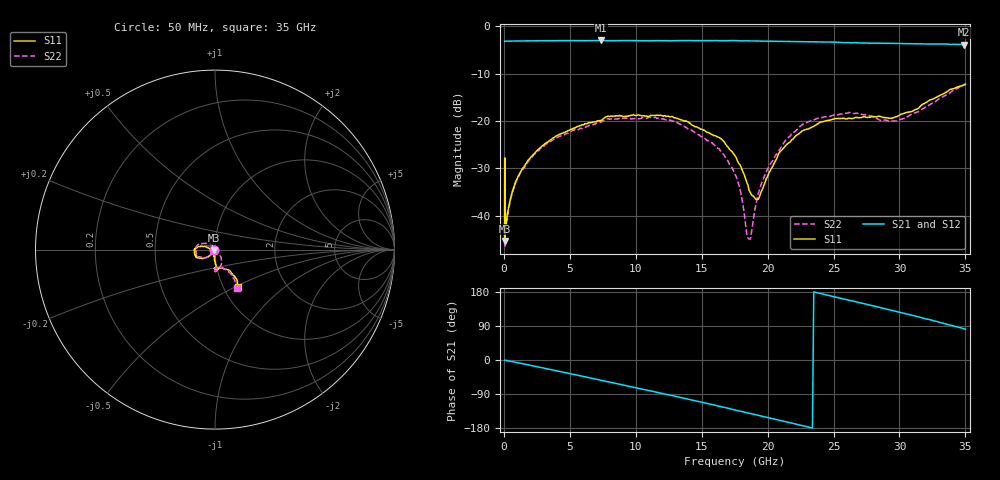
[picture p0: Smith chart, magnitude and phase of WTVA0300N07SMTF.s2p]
! 50 ohm 2-Port S-parameters measured by Modelithics Inc support@modelithics.com  Tampa, FL USA 813-866-6335 (February 2024)
! Smiths Interconnect,  3dB P/N: WTVA0300N07SMTF, Temperature: 25C
! Board: 10 mil Rogers 4350B, Mounting Pad Dimensions: Length: 15 mils, Width: 25 mils, Gap: 40 mils.
# Hz S MA R 50
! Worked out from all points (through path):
!   486 points, 50 MHz to 35 GHz, reference 50 ohm
!   highest |S21| = -2.97 dB at 7.35 GHz (marker M1); lowest = -3.8 dB at 34.9 GHz (marker M2)
!   group delay of S21, straight-line fit = 21.9 ps
!   lowest |S11| = -45.4 dB at 50 MHz (marker M3), VSWR 1.01, Z = 49.5 - j0.282 ohm
!   |S11| at or under -10 dB: start of sweep to end of sweep
!   |S22| runs from -46.5 to -12.2 dB; largest |S21 - S12| = 0.016
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5e7  0.005376 -148.1  0.6975 -0.4  0.6974 -0.4  0.004999 -168.1
8e7  0.006827 -143.7  0.6983 -0.5  0.6975 -0.5  0.004748 -157.2
9e7  0.008086 -161.6  0.6982 -0.6  0.6979 -0.6  0.006899 -158.3
5e8  0.01522 -130.1  0.6993 -3.3  0.699 -3.3  0.01473 -127.3
9e8  0.02285 -127.3  0.7018 -6.1  0.7019 -6.0  0.02237 -125.0
1.95e9  0.04015 -129.9  0.7035 -13.6  0.7034 -13.6  0.03912 -126.7
3.7e9  0.0658 -137.4  0.7066 -26.4  0.7063 -26.4  0.06275 -136.7
5.9e9  0.09124 -148.0  0.7064 -42.5  0.7063 -42.5  0.08326 -148.1
7.35e9  0.1013 -154.4  0.7106 -53.3  0.7105 -53.2  0.09724 -155.5
1.17e10  0.1149 -178.4  0.7067 -86.0  0.7064 -85.8  0.1074 174.1
1.58e10  0.07184 165.2  0.7072 -117.7  0.7075 -117.7  0.05848 142.6
1.76e10  0.04137 165.4  0.7085 -132.6  0.7084 -132.4  0.02614 119.4
1.86e10  0.01841 -176.9  0.7028 -140.5  0.702 -140.4  0.005632 34.1
1.92e10  0.01474 -135.7  0.7008 -145.4  0.7008 -145.3  0.01523 -29.8
2.01e10  0.02829 -97.7  0.6977 -152.6  0.6974 -152.3  0.03356 -47.4
2.12e10  0.05153 -92.9  0.6958 -161.5  0.6955 -161.3  0.05787 -53.0
2.34e10  0.08663 -86.4  0.6887 -179.5  0.689 -179.2  0.1012 -74.9
2.62e10  0.107 -91.9  0.6721 157.6  0.6719 157.7  0.1233 -88.5
2.92e10  0.1068 -75.5  0.663 132.9  0.6631 133.4  0.09943 -84.4
3.19e10  0.1534 -54.7  0.6515 109.3  0.6513 110.5  0.1377 -58.7
3.49e10  0.2406 -57.5  0.6432 82.4  0.643 82.7  0.2424 -59.9
3.5e10  0.2451 -57.8  0.6435 81.5  0.643 81.8  0.2466 -60.5
